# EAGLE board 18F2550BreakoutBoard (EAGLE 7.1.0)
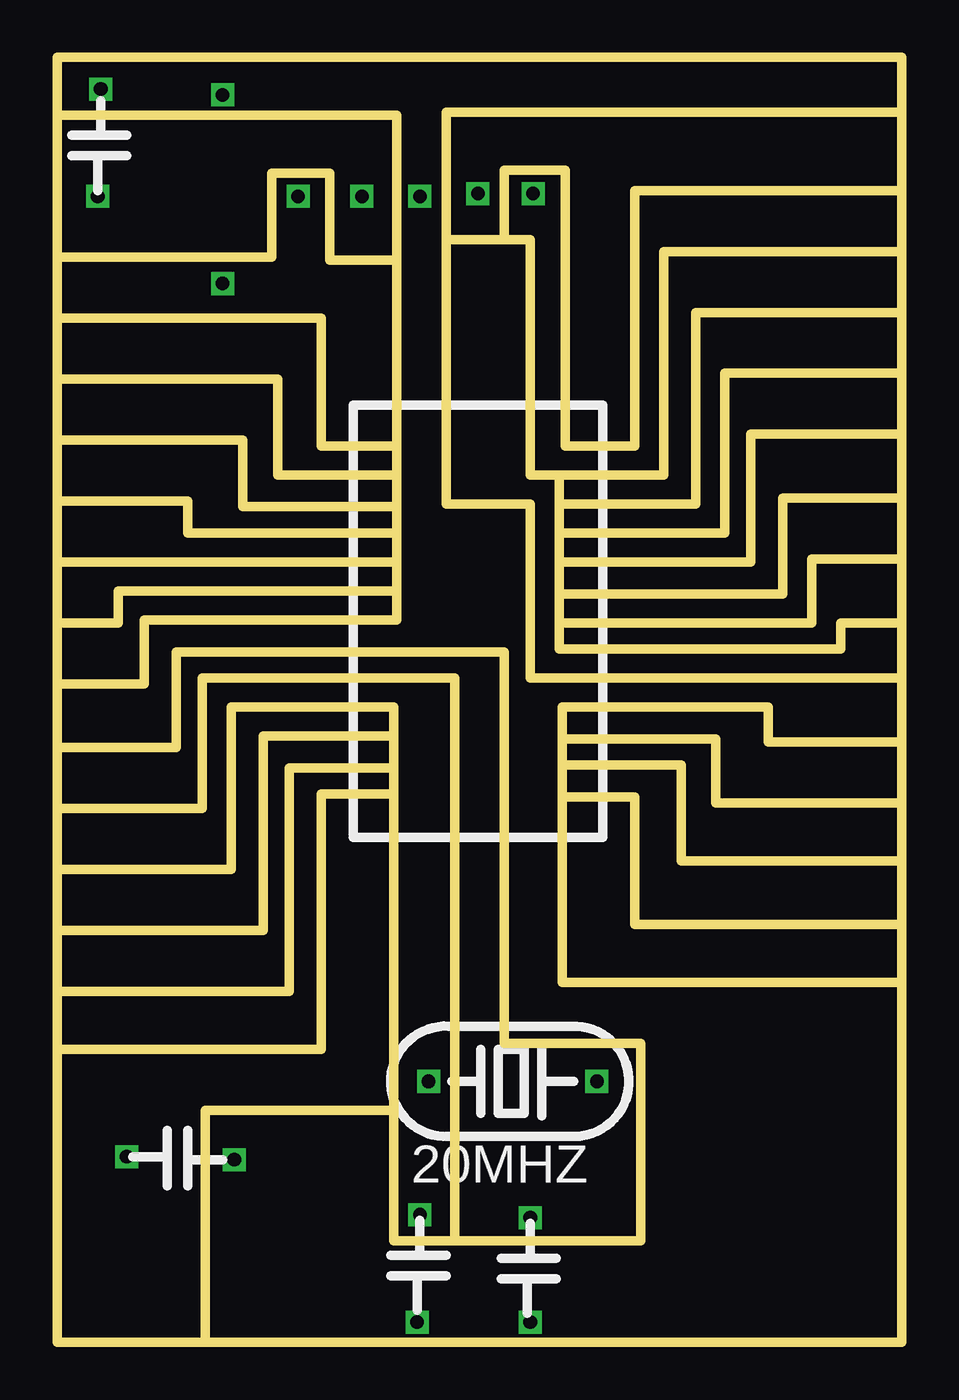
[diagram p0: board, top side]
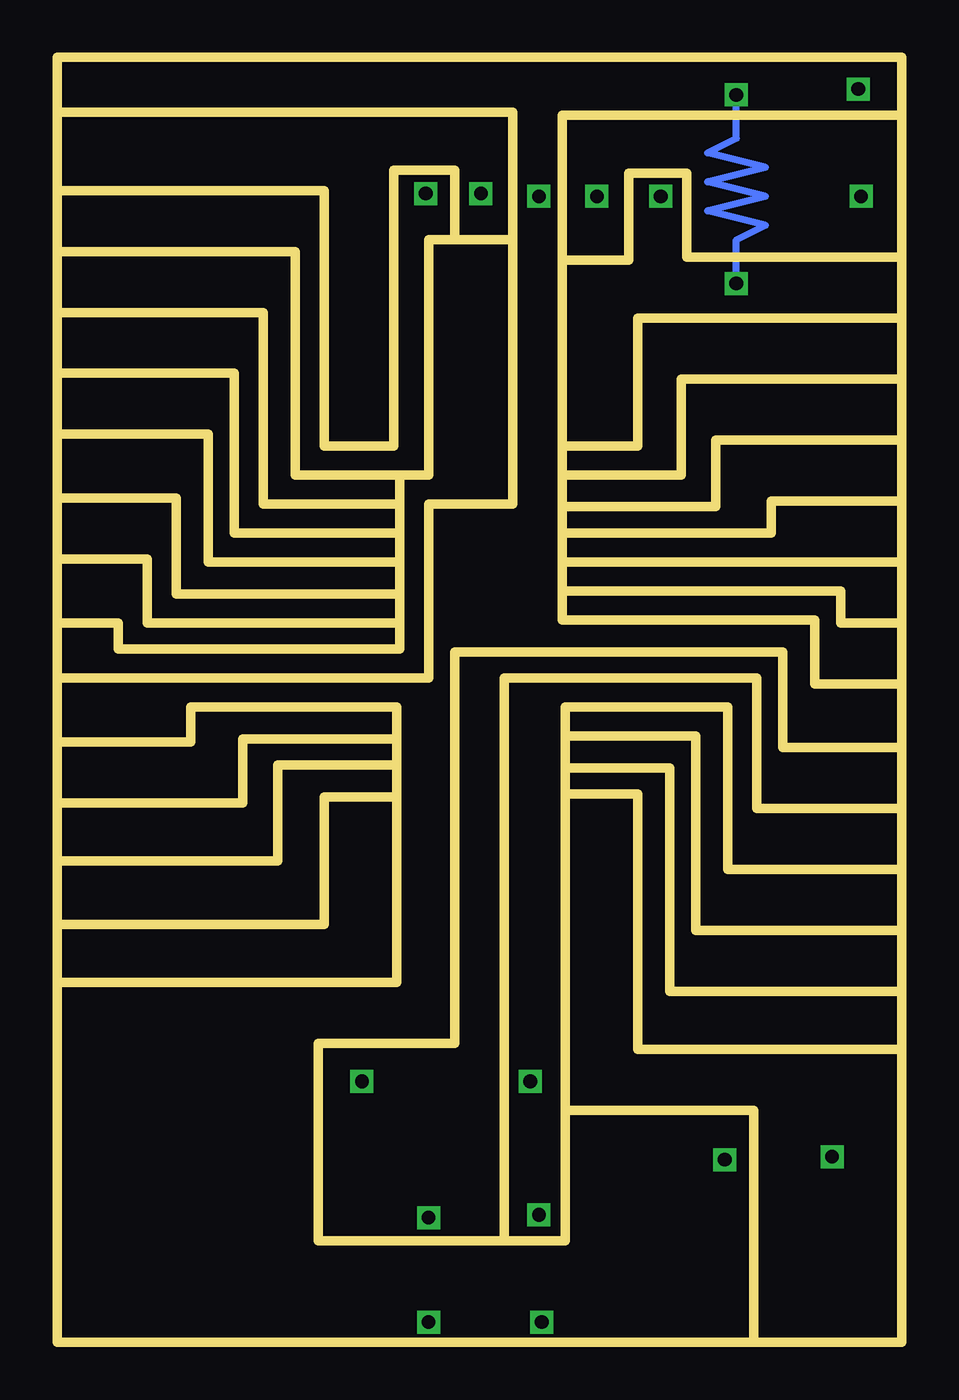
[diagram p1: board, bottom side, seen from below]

Size 36.96 x 56.26 mm. Coordinates in mm from the lower left corner, seen from the top.
Outline: 164 segments
Copper layers (1*16): Top 0.035mm / dielectric 1.5mm / Bottom 0.035mm
Design rules "default *": minimum track width 10mil, minimum drill 24mil, track to track 1mil, track to pad 1mil, pad to pad 8mil, via to via 8mil, smd to smd 8mil, copper to edge 10mil, drill to drill 1mil, minimum pad ring 10mil, minimum via ring 8mil, stop-mask expansion 4mil, vias tented up to drill 0mil, thermal gap 10mil

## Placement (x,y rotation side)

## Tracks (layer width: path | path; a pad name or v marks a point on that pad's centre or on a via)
S$1  (via drill 0.6)
  other vias: 10.54,50.16
S$2  (via drill 0.6)
  other vias: 13.34,50.16
S$3  (via drill 0.6)
  other vias: 15.88,50.16
S$4  (via drill 0.6)
  other vias: 18.41,50.29
S$5  (via drill 0.6)
  other vias: 20.83,50.29
S$6  (via drill 0.6)
  other vias: 16.26,11.43
S$7  (via drill 0.6)
  other vias: 23.62,11.43
S$8  (via drill 0.6)
  other vias: 15.88,5.59
S$9  (via drill 0.6)
  other vias: 20.7,5.46
S$10  (via drill 0.6)
  other vias: 20.7,0.89
S$11  (via drill 0.6)
  other vias: 15.75,0.89
S$12  (via drill 0.6)
  other vias: 3.05,8.13
S$13  (via drill 0.6)
  other vias: 7.75,8
S$14  (via drill 0.6)
  other vias: 1.78,50.16
S$15  (via drill 0.6)
  other vias: 1.91,54.86
S$19  (via drill 0.6)
  Bottom 0.305: v7.24,46.36 7.24,48.26 5.97,48.9 8.51,49.53 5.97,50.16 8.51,50.8 5.97,51.44 8.51,52.07 7.24,52.71 v7.24,54.61

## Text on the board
Unrouted: PIC PROGRAMMER | MCLR | VDD | VSS | PGD | PGC | 470nf | PGD | 10k | PGC | MCLR | RB5 | RA0 | RB4 | RA1 | RB3 | RA2 | RB2 | RA3 | RB1 | RA4 | RB0 | RA5 | VDD | VSS | VSS | OSC1 | RC7 | OSC2 | RC6 | RC0 | D+ | RC1 | D- | RC2 | VUSB | 470nf | 22pf | 22pf
tPlace: 20MHZ
200bmp: C:/Users/kramerr/Desktop/eagle scripts/BottomEnhanced.bmp | C:/Users/kramerr/Desktop/eagle scripts/BottomEnhanced.bmp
